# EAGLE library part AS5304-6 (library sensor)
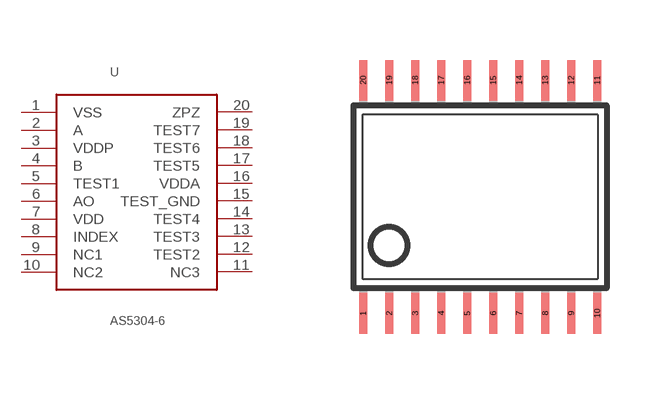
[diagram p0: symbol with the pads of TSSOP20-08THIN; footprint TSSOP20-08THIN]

Designator prefix -

## AS5304-6  [TSSOP20-08THIN]
1  VSS
2  A
3  VDDP
4  B
5  TEST1
6  AO
7  VDD
8  INDEX
9  NC1
10  NC2
11  NC3
12  TEST2
13  TEST3
14  TEST4
15  TEST_GND
16  VDDA
17  TEST5
18  TEST6
19  TEST7
20  ZPZ

## Footprint TSSOP20-08THIN (pad centres in mm)
Thin Shrink Small Outline Plastic 20 MAX3223-MAX3243.pdf
smd 0.203 x 1.016: 1 -2.925,-2.918; 2 -2.275,-2.918; 3 -1.625,-2.918; 4 -0.975,-2.918; 5 -0.325,-2.918; 6 0.325,-2.918; 7 0.975,-2.918; 8 1.625,-2.918; 9 2.275,-2.918; 10 2.925,-2.918; 11 2.925,2.918; 12 2.275,2.918; 13 1.625,2.918; 14 0.975,2.918; 15 0.325,2.918; 16 -0.325,2.918; 17 -0.975,2.918; 18 -1.625,2.918; 19 -2.275,2.918; 20 -2.925,2.918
